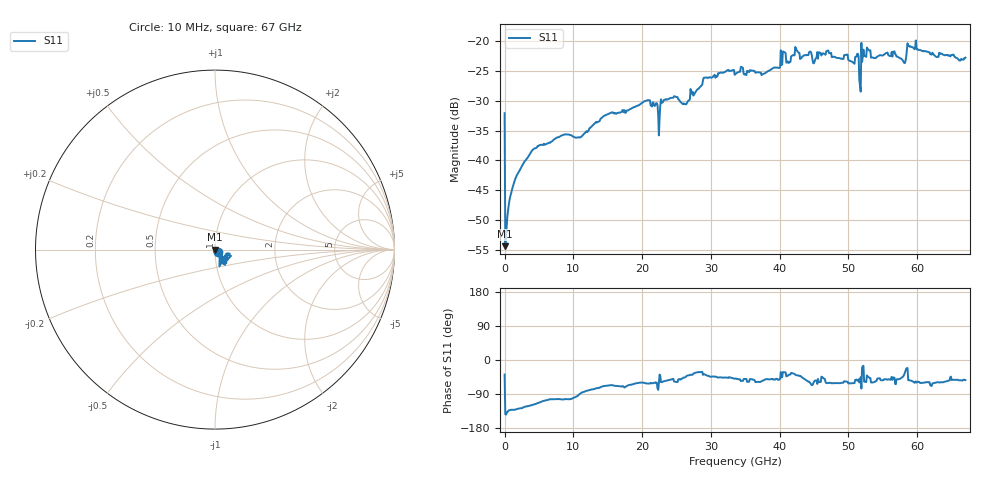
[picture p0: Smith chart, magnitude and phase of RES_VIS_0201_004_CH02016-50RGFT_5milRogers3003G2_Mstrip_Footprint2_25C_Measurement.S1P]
! 50 Ohm 1-port S-parameter data measured by Modelithics Inc.  support@modelithics.com 813-866-6335  Tampa FL USA
! Vishay, 0201, 50 Ohm P/N: CH02016-50RGFT, Model name:RES_VIS_0201_004, Temperature: 25C,
! Substrate: 5-mil Rogers 3003G2 Microstrip, Footprint2, substrate thickness, H=0.127mm, Dielectric constant, Er=3.07
! PCB Mounting Pad Footprint#2: Pad width, PadW=0.450mm , Pad length, PadL=0.200mm , Pad gap, PadG (edge-to-edge)=0.150mm, GND PADL=0.750mm, GND PADW=1.652mm, VIAD=0.152mm
# Hz S MA R 50
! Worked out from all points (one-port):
!   670 points, 10 MHz to 67 GHz, reference 50 ohm
!   lowest |S11| = -54.4 dB at 110.1 MHz (marker M1), VSWR 1.00, Z = 49.8 - j0.114 ohm
!   |S11| at or under -10 dB: start of sweep to end of sweep
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1e7  0.02484 -38.5
1.101345e8  0.001912 -143.1
4.105381e8  0.0034 -136.6
1.211614e9  0.00604 -131.4
2.813767e9  0.009577 -124.4
4.315785e9  0.01253 -117.0
8.4213e9  0.01627 -104.2
1.10248e10  0.01562 -88.6
1.68326e10  0.02523 -69.5
2.083798e10  0.03197 -62.2
2.234e10  0.02412 -78.8
2.304094e10  0.03082 -57.1
2.514377e10  0.03387 -58.5
2.624525e10  0.02958 -45.7
2.914915e10  0.04936 -38.4
3.355507e10  0.05281 -48.9
3.766058e10  0.05315 -53.7
4.196637e10  0.07638 -35.1
4.507054e10  0.06721 -54.9
4.707323e10  0.08327 -60.8
5.027753e10  0.06803 -61.8
5.117874e10  0.07404 -51.7
5.177955e10  0.0377 -45.3
5.218009e10  0.0847 -15.3
5.288103e10  0.08479 -45.0
5.798789e10  0.06726 -42.8
5.868883e10  0.09049 -53.3
6.7e10  0.07254 -53.0
